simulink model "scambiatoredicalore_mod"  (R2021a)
settings: Solver=FixedStepAuto  StartTime=0.0  StopTime=10000  FixedStep=Tsim  MaxStep=1  RelTol=1e-3
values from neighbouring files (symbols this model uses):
  ca = 4178    [scambiatoredicalore_dati.m]    (also in scambiatoremodelloTD.m)
  cb = 2131    [scambiatoredicalore_dati.m]    (also in scambiatoremodelloTD.m)
  ma = rhoa*pi*Di^2/4*L    (= 38.4179965995)    [scambiatoredicalore_dati.m]    (also in scambiatoremodelloTD.m)
  mb = rhob*pi*(Dan^2-De^2)/4*L    (= 72.0857488137)    [scambiatoredicalore_dati.m]    (also in scambiatoremodelloTD.m)
  Rba = Ri+Re+Rparete    [scambiatoredicalore_dati.m]    (also in scambiatoremodelloTD.m)
  Ta0 = 35    [scambiatoremodelloTD.m]
  Tain = 30    [scambiatoredicalore_dati.m]    (also in scambiatoremodelloTD.m)
  Tb0 = 55    [scambiatoremodelloTD.m]
  Tbin = 100    [scambiatoredicalore_dati.m]    (also in scambiatoremodelloTD.m)
  wa = 0.2    [scambiatoredicalore_dati.m]    (also in scambiatoremodelloTD.m)
  wb = 0.1    [scambiatoredicalore_dati.m]    (also in scambiatoremodelloTD.m)

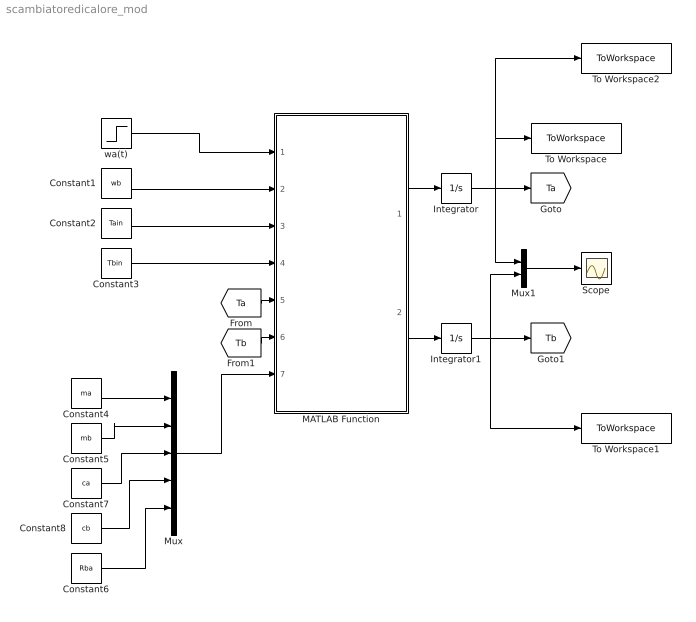
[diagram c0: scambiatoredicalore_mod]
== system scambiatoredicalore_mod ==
  Constant1 : Constant  Value=wb
  Constant2 : Constant  Value=Tain
  Constant3 : Constant  Value=Tbin
  Constant4 : Constant  Value=ma
  Constant5 : Constant  Value=mb
  Constant6 : Constant  Value=Rba
  Constant7 : Constant  Value=ca
  Constant8 : Constant  Value=cb
  Integrator : Integrator  InitialCondition=Ta0
  Integrator1 : Integrator  InitialCondition=Tb0
  MATLAB Function : MATLAB Function  TreatAsAtomicUnit=on
  Mux : Mux  Inputs=5
  Mux1 : Mux  Inputs=2
  Scope : Scope
  To Workspace : ToWorkspace  VariableName=simout  SaveFormat=Timeseries  SampleTime=-1
  To Workspace1 : ToWorkspace  VariableName=Tbmod  SaveFormat=Timeseries  SampleTime=-1
  To Workspace2 : ToWorkspace  VariableName=Tamod  SaveFormat=Timeseries  SampleTime=-1
  wa(t) : Step  Time=5000  Before=wa  After=2*wa  SampleTime=0
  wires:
  MATLAB Function/1(Tadot) -> Integrator/1
  MATLAB Function/2(Tbdot) -> Integrator1/1
  Integrator/1 -> [Ta], To Workspace2/1, To Workspace/1, Mux1/1
  Integrator1/1 -> To Workspace1/1, Mux1/2, [Tb]
  [Ta] -> MATLAB Function/5(Ta)
  [Tb] -> MATLAB Function/6(Tb)
  wa(t)/1 -> MATLAB Function/1(wa)
  Constant1/1 -> MATLAB Function/2(wb)
  Constant2/1 -> MATLAB Function/3(Tain)
  Constant3/1 -> MATLAB Function/4(Tbin)
  Constant4/1 -> Mux/1
  Constant5/1 -> Mux/2
  Mux/1 -> MATLAB Function/7(par)
  Constant7/1 -> Mux/3
  Constant8/1 -> Mux/4
  Constant6/1 -> Mux/5
  Mux1/1 -> Scope/1

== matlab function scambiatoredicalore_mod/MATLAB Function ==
function [Tadot,Tbdot] = fcn(wa,wb,Tain,Tbin,Ta,Tb,par)

ma=par(1);
mb=par(2);
ca=par(3);
cb=par(4);
Rba=par(5);

DT1=Tbin-Ta;
DT2=Tb-Tain;

Tadot =  1/ma*wa*(Tain-Ta)+1/(Rba*ma*ca)*(DT1-DT2)/log(DT1/DT2);
Tbdot =  1/mb*wb*(Tbin-Tb)-1/(Rba*mb*cb)*(DT1-DT2)/log(DT1/DT2);
